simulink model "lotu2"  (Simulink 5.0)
settings: Solver=ode45  StartTime=0.0  StopTime=10.0  RelTol=1e-3

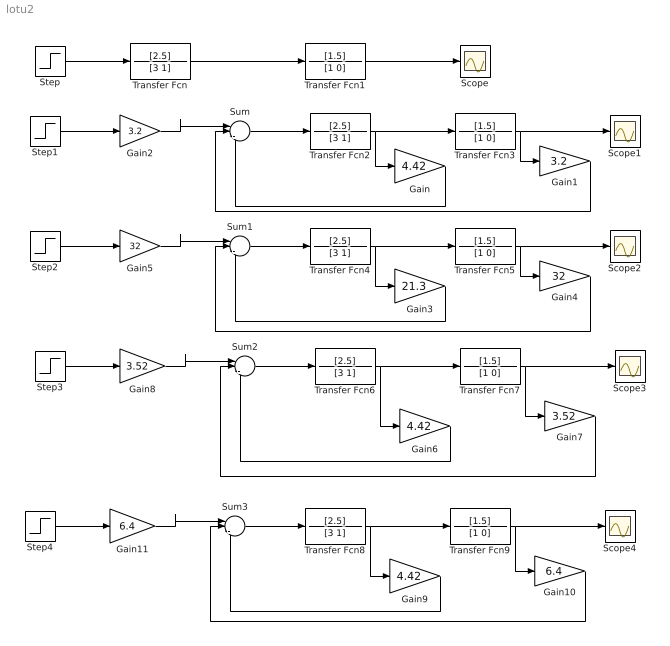
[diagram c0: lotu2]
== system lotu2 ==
  Gain : Gain  Gain=4.42
  Gain1 : Gain  Gain=3.2
  Gain10 : Gain  Gain=6.4
  Gain11 : Gain  Gain=6.4
  Gain2 : Gain  Gain=3.2
  Gain3 : Gain  Gain=21.3
  Gain4 : Gain  Gain=32
  Gain5 : Gain  Gain=32
  Gain6 : Gain  Gain=4.42
  Gain7 : Gain  Gain=3.52
  Gain8 : Gain  Gain=3.52
  Gain9 : Gain  Gain=4.42
  Scope{,1..4} (5 alike) : Scope
  Step{,1..4} (5 alike) : Step  Time=0  SampleTime=0
  Sum{,1..3} (4 alike) : Sum  Inputs=|+--
  Transfer Fcn{,2,4,6,8} (5 alike) : TransferFcn  Numerator=[2.5]  Denominator=[3 1]
  Transfer Fcn{1,3,5,7,9} (5 alike) : TransferFcn  Numerator=[1.5]  Denominator=[1 0]
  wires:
  Step/1 -> Transfer Fcn/1
  Transfer Fcn/1 -> Transfer Fcn1/1
  Transfer Fcn1/1 -> Scope/1
  Transfer Fcn2/1 -> Transfer Fcn3/1, Gain/1
  Transfer Fcn3/1 -> Gain1/1, Scope1/1
  Sum/1 -> Transfer Fcn2/1
  Step1/1 -> Gain2/1
  Gain/1 -> Sum/3
  Gain1/1 -> Sum/2
  Gain2/1 -> Sum/1
  Transfer Fcn4/1 -> Transfer Fcn5/1, Gain3/1
  Transfer Fcn5/1 -> Gain4/1, Scope2/1
  Sum1/1 -> Transfer Fcn4/1
  Step2/1 -> Gain5/1
  Gain3/1 -> Sum1/3
  Gain4/1 -> Sum1/2
  Gain5/1 -> Sum1/1
  Transfer Fcn6/1 -> Transfer Fcn7/1, Gain6/1
  Transfer Fcn7/1 -> Gain7/1, Scope3/1
  Sum2/1 -> Transfer Fcn6/1
  Step3/1 -> Gain8/1
  Gain6/1 -> Sum2/3
  Gain7/1 -> Sum2/2
  Gain8/1 -> Sum2/1
  Transfer Fcn8/1 -> Transfer Fcn9/1, Gain9/1
  Transfer Fcn9/1 -> Gain10/1, Scope4/1
  Sum3/1 -> Transfer Fcn8/1
  Step4/1 -> Gain11/1
  Gain9/1 -> Sum3/3
  Gain10/1 -> Sum3/2
  Gain11/1 -> Sum3/1
